(* Logix 5000 AddOnInstructionDefinition export Banner_K50Z_Param_v4; software revision 33.00 *)

TYPE Banner_IOL_Port_v4 :   // UDT that has all of the data items necessary to communicate with a specific Port on a IO-Link Master
STRUCT
   Port_Controlled : INT;   // Each bit represents a port on an IO-Link Master. Set to 1 to tell AOI to control that port.
   Port_Activate : INT;   // Each bit represents a port on an IO-Link Master. When ON that port will process any commands in queue.
   Port_Read : INT;   // Each bit represents a port on an IO-Link Master. Used to determine when device AOI has requested a Read command.
   Port_Write : INT;   // Each bit represents a port on an IO-Link Master. Used to determine when device AOI has requested a Write command.
   Port_RW_Complete : INT;   // Each bit represents a port on an IO-Link Master. Tells device AOI that Read or Write request has been completed.
   Port_Device_Read : INT;
   Data_Transfer : SINT[190];   // Array to transfer data from IO-Master to device AOIs.
END_STRUCT
END_TYPE

TYPE Banner_K50Z_BDC_v4 :   // All of the BDC data for channels 1 and 2.
STRUCT
   SP1 : DINT;   // Switchpoint.
   SP2 : DINT;   // In 2pt window mode, defines the second switching point. In other modes, SP2 is unused and must be 0.
   Switchpoint_Logic : SINT;   // 0 = Light operate, 1 = Dark operate
   BDC_Mode : INT;   // 1 = 1pt Object Set, 128 = 2pt static BGS, 129 = 2pt Window FGS, 130 = 1pt Window FGS, 131 = Dual Mode.
   Hysteresis : INT;   // A value of 0 will result in automatically calculated hysteresis.
   Delay_Mode : SINT;   // 0 = Disabled, 1 = On Off Delay, 2 = Oneshot.
   Delay_Time_On_Oneshot : DINT;   // 0 to 90000. On delay and oneshot time.
   Delay_Time_Off : DINT;   // 0 to 90000. Off delay only.
   Teach_Offset : SINT;   // 0 = Auto, 1 = User Selected
   User_Teach_Offset : DINT;   // In Object Set or Window (FGS) mode this value can be either positive or negative. In all other modes must be zero.
END_STRUCT
END_TYPE

TYPE Banner_K50Z_Pulse_Freq_v4 :
STRUCT
   Near_Freq : DINT;   // 1 to 100000 in Hz
   Far_Freq : DINT;   // 1 to 100000 in Hz
   SP1 : DINT;   // Switchpoint
   SP2 : DINT;   // In 2pt Window FGS teach, define the second switching point. In other modes SP2 should be zero.
   Pulse_Freq_LOS : DINT;   // Default value of 50. This is the Hz that the units outputs when a Loss of Signal occurs.
END_STRUCT
END_TYPE

TYPE Banner_K50Z_RD_v4 :   // UDT that stores the Write Data for a K50Z.
STRUCT
   Master_Cycle_Time : INT;
   Min_Cycle_Time : INT;
   M_Sequence_Capability : INT;
   IO_Link_Version_ID : INT;
   Process_Data_Input_Length : INT;
   Process_Data_Output_Length : INT;
   Combined_Vendor_ID : DINT;   // IO-Link Vendor ID
   Vendor_ID1 : INT;
   Vendor_ID2 : INT;
   Combined_Device_ID : DINT;   // IO-Link Device ID
   Device_ID1 : INT;
   Device_ID2 : INT;
   Device_ID3 : INT;
   Serial_Number : STRING;
   Teach_State : SINT;   // 0=Idle, 1=SP1 Success, 4=Wait for Command, 5=Busy, 7=Error.
   SP1_TP1 : SINT;
   SP1_TP2 : SINT;
   Measurement_Z1 : DINT;
   Excess_Gain_Z1 : DINT;   // Amount of singal measured over the minimum threshold.
   Stability_Z1 : SINT;   // 0=No target exists, 1=Marginal signal, 2=Stable.
   Measurement_Z2 : DINT;
   Excess_Gain_Z2 : DINT;   // Amount of singal measured over the minimum threshold.
   Stability_Z2 : SINT;   // 0=No target exists, 1=Marginal signal, 2=Stable.
   Emitter_Status : SINT;   // 0 = Active, 1 = Inactive
   Temperature : DINT;   // Internal temperature measurement for the device.
   Last_Taught_Temperature : DINT;   // Internal Temperature the last time device was taught.
   MDC_Lower_Limit : DINT;
   MDC_Upper_Limit : DINT;
   MDC_Unit : INT;
   MDC_Scale : SINT;
END_STRUCT
END_TYPE

TYPE Banner_K50Z_v4 :   // All of the parameters for a K50Z.
STRUCT
   Initial_Global_Read : BOOL;   // Determines if all of the IO-Link data has been read into the PLC yet
   Command : INT;   // Value placed in here will activate a read or write to a specifc IO-Link Index
   Read : Banner_K50Z_RD_v4;   // Read Only Data
   Write : Banner_K50Z_WD_v4;   // Write Data
   Archive : Banner_K50Z_WD_v4;   // Archive Data
   Reset : BOOL;   // Resets AOI. This will force a complete parameter read of the sensor.
END_STRUCT
END_TYPE

TYPE Banner_K50Z_WD_v4 :   // UDT that stores the Write Data for a K50Z.
STRUCT
   System_Command : INT;   // See IODD file for list of commands that can be activated via the System Command interface
   Parameter_Access_Lock : SINT;   // Write access to all parameters is prohibited while value is 1. Only this parameter can be adjusted when value is 1.
   Data_Storage_Lock : SINT;   // Automatic data storage is disabled when this value is equal to 1. Read access is not affected.
   Local_Parameterization_Lock : SINT;   // Parameterization via local control elements on device is disabled.
   Local_User_Interface_Lock : SINT;   // Operation of local user interface is disabled.
   Teach_Channel : SINT;   // 0 = Default, 1 = BDC1, 2 = BDC2
   Response_Speed : SINT;   // 0 = Speed 0, 1 = Speed 1, 2 = Speed 2, 3 = Speed 3
   Remote_Input_Mode : SINT;   // 0 = Remote Teach Input, 1 = Emitter On, 2 = Emitter Off
   Secondary_Output_Mode : SINT;   // 0 = Independent Output, 1 = Complementary Output, 2 = Pulse Frequency Output
   IOL_Filter_Time : INT;   // Time to average IOl process data measurement between updates
   Include_Binary : SINT;   // 0 = Include, 1 = Don't Include, 2= Measurement Device
   Measurement_1 : SINT;   // 0 = Disabled, 1 = Excess Gain Z1, 2 = Excess Gain Z2, 3 = Excess Gain / 10 Z1, 4 = Excess Gain / 10 Z2, 5 = Measurement Z1, 6 = Measurement Z2.
   Measurement_2 : SINT;   // 0 = Disabled, 1 = Excess Gain Z1, 2 = Excess Gain Z2, 3 = Excess Gain / 10 Z1, 4 = Excess Gain / 10 Z2, 5 = Measurement Z1, 6 = Measurement Z2.
   Digital_Measuring_Sensor_Zone_Selection : SINT;   // 0=Zone 1, 1=Zone2
   BDC : Banner_K50Z_BDC_v4[3];
   Pulse_Freq : Banner_K50Z_Pulse_Freq_v4;
END_STRUCT
END_TYPE

ADD_ON_INSTRUCTION Banner_K50Z_Param_v4   (* revision 4.1, vendor Banner Engineering *)
// AOI to read and write parameter data to an IO-Link K50Z.
VAR_IN_OUT
   K50Z : Banner_K50Z_v4; {required}
   Port_Data : Banner_IOL_Port_v4; {required}
END_VAR
VAR_INPUT
   Port : DINT; {required}
END_VAR
VAR
   Local_Control : DINT; {access None}
   Global_Read_Command_Value : INT; {access None}
   Global_Write_Command_Value : INT; {access None}
   Command_Being_Processed : BOOL; {access None}
   Update_Archive : BOOL; {access None}
   Index_Write_Inprocess : INT; {access None}
   Index_Write_Control : INT; {access None}
   Inprocess_Index : DINT; {access None}
END_VAR

ROUTINE Logic   (* ladder *)
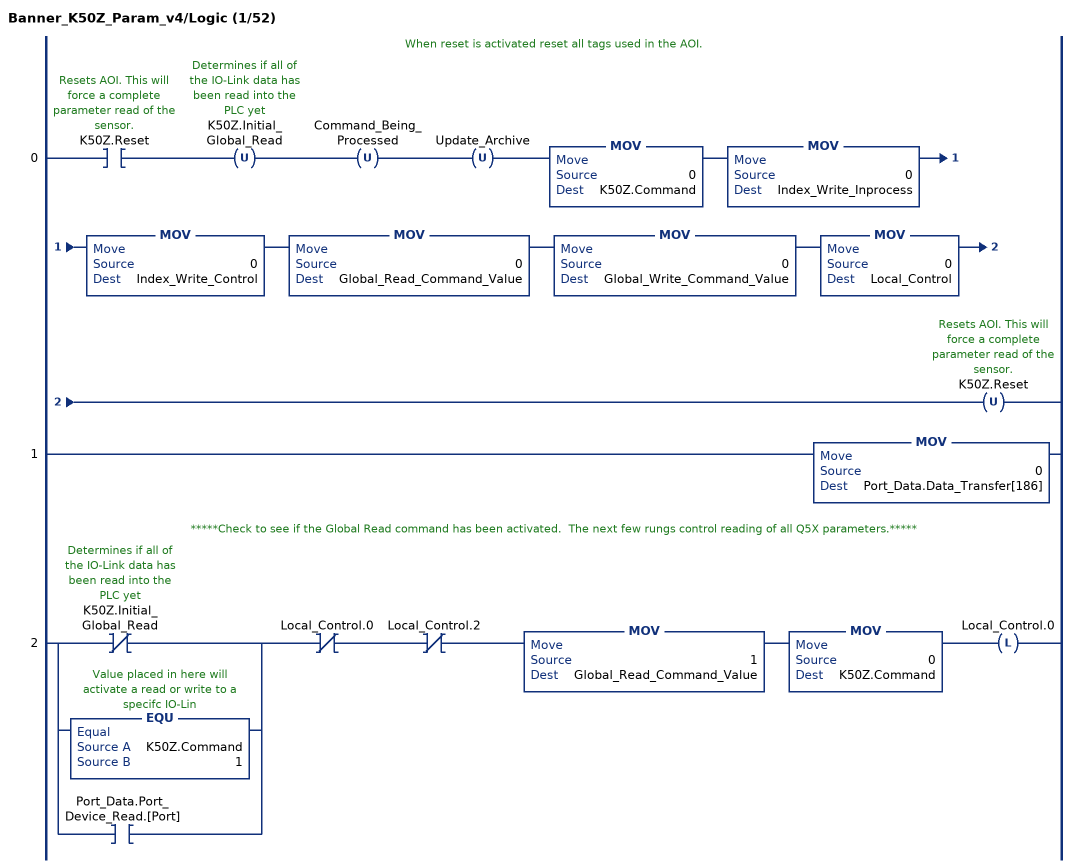
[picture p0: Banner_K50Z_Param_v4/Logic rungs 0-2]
   // When reset is activated reset all tags used in the AOI.
   0: XIC(K50Z.Reset)OTU(K50Z.Initial_Global_Read)OTU(Command_Being_Processed)OTU(Update_Archive)MOV(0,K50Z.Command)MOV(0,Index_Write_Inprocess)MOV(0,Index_Write_Control)MOV(0,Global_Read_Command_Value)MOV(0,Global_Write_Command_Value)MOV(0,Local_Control)OTU(K50Z.Reset);
   1: MOV(0,Port_Data.Data_Transfer[186]);
   // *****Check to see if the Global Read command has been activated.  The next few rungs control reading of all Q5X parameters.*****
   2: [XIO(K50Z.Initial_Global_Read) ,EQU(K50Z.Command,1) ,XIC(Port_Data.Port_Device_Read.[Port]) ]XIO(Local_Control.0)XIO(Local_Control.2)MOV(1,Global_Read_Command_Value)MOV(0,K50Z.Command)OTL(Local_Control.0);
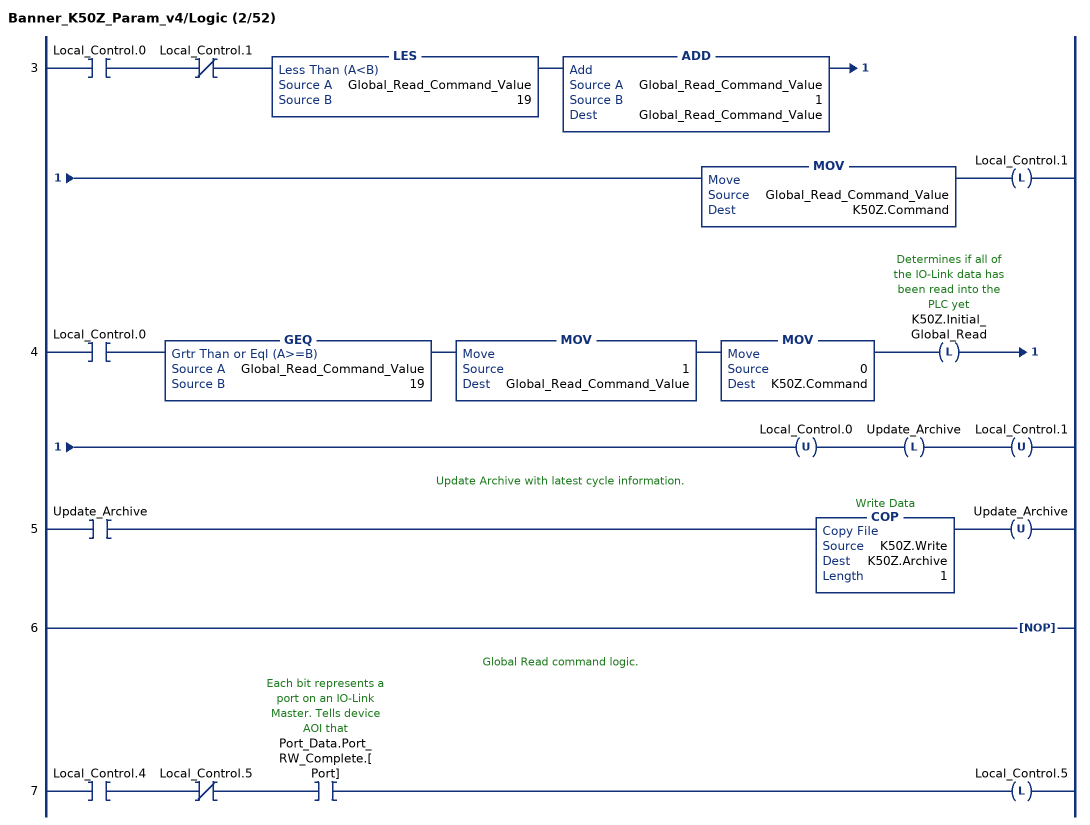
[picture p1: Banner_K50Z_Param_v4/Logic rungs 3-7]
   3: XIC(Local_Control.0)XIO(Local_Control.1)LES(Global_Read_Command_Value,19)ADD(Global_Read_Command_Value,1,Global_Read_Command_Value)MOV(Global_Read_Command_Value,K50Z.Command)OTL(Local_Control.1);
   4: XIC(Local_Control.0)GEQ(Global_Read_Command_Value,19)MOV(1,Global_Read_Command_Value)MOV(0,K50Z.Command)OTL(K50Z.Initial_Global_Read)OTU(Local_Control.0)OTL(Update_Archive)OTU(Local_Control.1);
   // Update Archive with latest cycle information.
   5: XIC(Update_Archive)COP(K50Z.Write,K50Z.Archive,1)OTU(Update_Archive);
   6: NOP();
   // Global Read command logic.
   7: XIC(Local_Control.4)XIO(Local_Control.5)XIC(Port_Data.Port_RW_Complete.[Port])OTL(Local_Control.5);
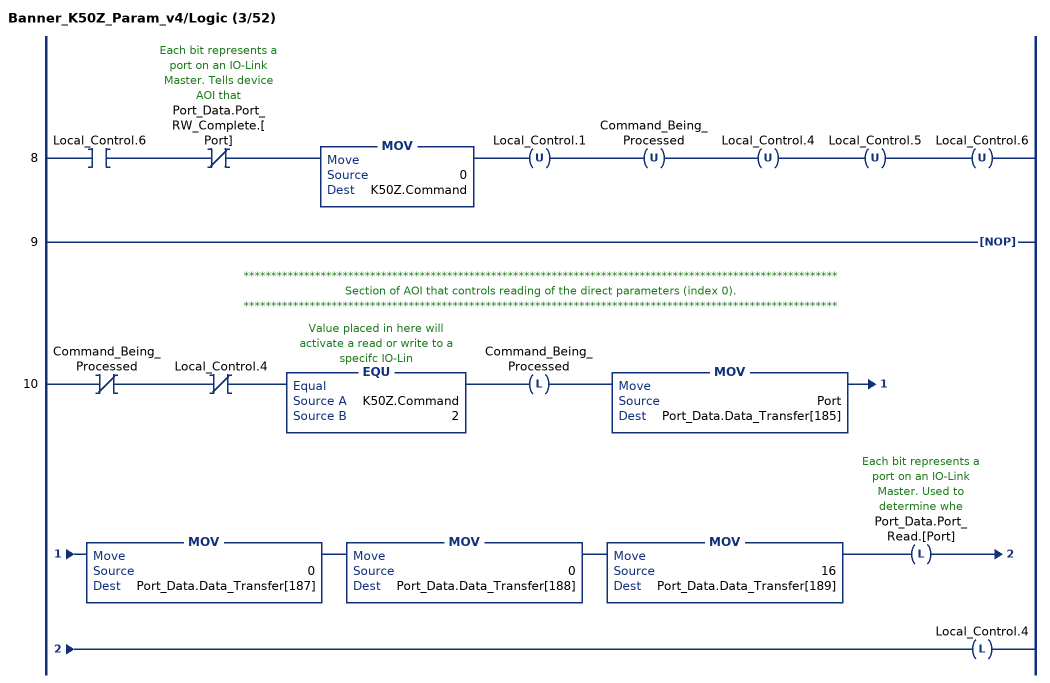
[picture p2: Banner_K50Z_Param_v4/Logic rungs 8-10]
   8: XIC(Local_Control.6)XIO(Port_Data.Port_RW_Complete.[Port])MOV(0,K50Z.Command)OTU(Local_Control.1)OTU(Command_Being_Processed)OTU(Local_Control.4)OTU(Local_Control.5)OTU(Local_Control.6);
   9: NOP();
   // ************************************************************************************************************
   // Section of AOI that controls reading of the direct parameters (index 0).
   // ************************************************************************************************************
   10: XIO(Command_Being_Processed)XIO(Local_Control.4)EQU(K50Z.Command,2)OTL(Command_Being_Processed)MOV(Port,Port_Data.Data_Transfer[185])MOV(0,Port_Data.Data_Transfer[187])MOV(0,Port_Data.Data_Transfer[188])MOV(16,Port_Data.Data_Transfer[189])OTL(Port_Data.Port_Read.[Port])OTL(Local_Control.4);
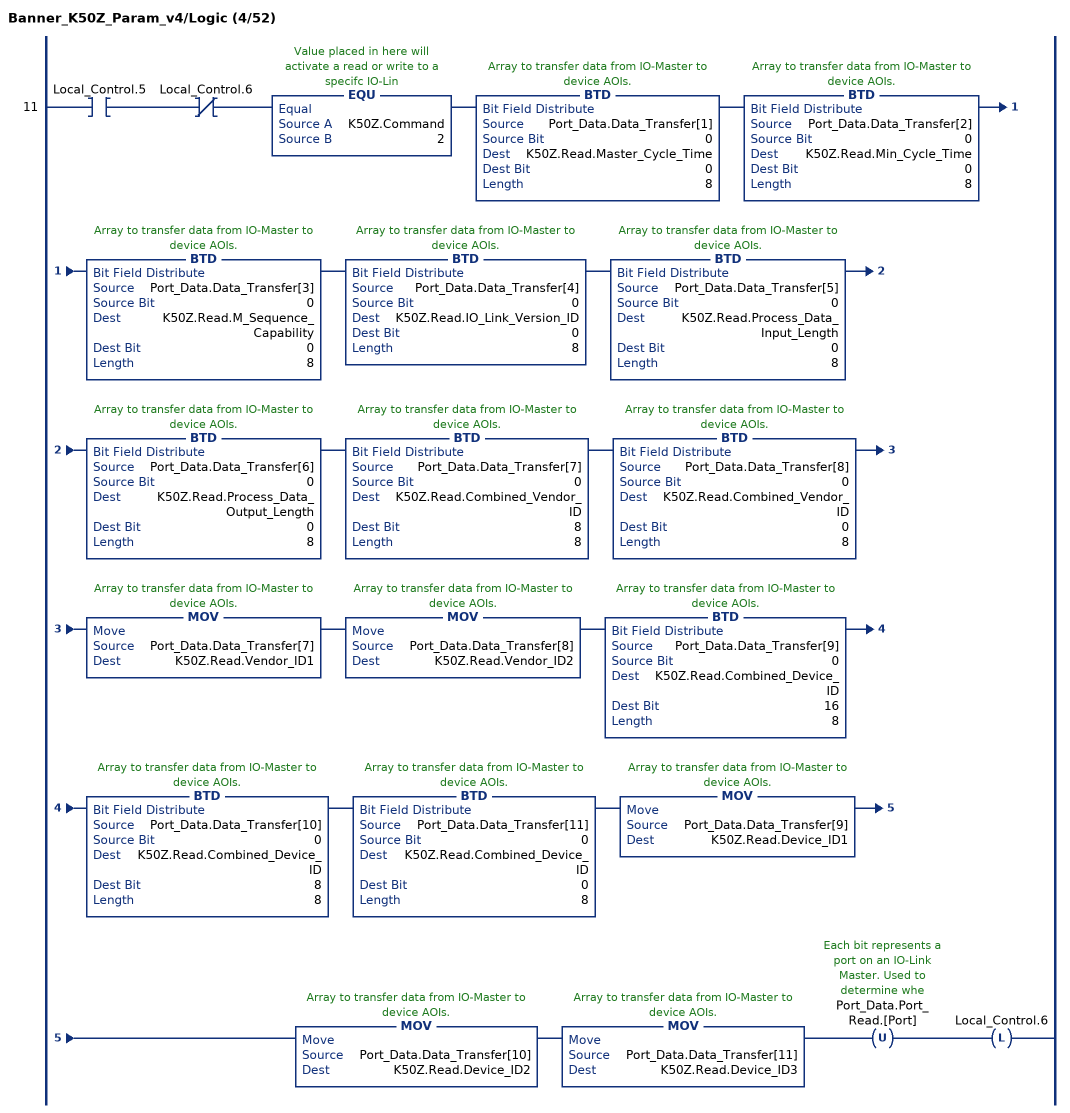
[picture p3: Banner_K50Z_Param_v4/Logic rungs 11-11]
   11: XIC(Local_Control.5)XIO(Local_Control.6)EQU(K50Z.Command,2)BTD(Port_Data.Data_Transfer[1],0,K50Z.Read.Master_Cycle_Time,0,8)BTD(Port_Data.Data_Transfer[2],0,K50Z.Read.Min_Cycle_Time,0,8)BTD(Port_Data.Data_Transfer[3],0,K50Z.Read.M_Sequence_Capability,0,8)BTD(Port_Data.Data_Transfer[4],0,K50Z.Read.IO_Link_Version_ID,0,8)BTD(Port_Data.Data_Transfer[5],0,K50Z.Read.Process_Data_Input_Length,0,8)BTD(Port_Data.Data_Transfer[6],0,K50Z.Read.Process_Data_Output_Length,0,8)BTD(Port_Data.Data_Transfer[7],0,K50Z.Read.Combined_Vendor_ID,8,8)BTD(Port_Data.Data_Transfer[8],0,K50Z.Read.Combined_Vendor_ID,0,8)MOV(Port_Data.Data_Transfer[7],K50Z.Read.Vendor_ID1)MOV(Port_Data.Data_Transfer[8],K50Z.Read.Vendor_ID2)BTD(Port_Data.Data_Transfer[9],0,K50Z.Read.Combined_Device_ID,16,8)BTD(Port_Data.Data_Transfer[10],0,K50Z.Read.Combined_Device_ID,8,8)BTD(Port_Data.Data_Transfer[11],0,K50Z.Read.Combined_Device_ID,0,8)MOV(Port_Data.Data_Transfer[9],K50Z.Read.Device_ID1)MOV(Port_Data.Data_Transfer[10],K50Z.Read.Device_ID2)MOV(Port_Data.Data_Transfer[11],K50Z.Read.Device_ID3)OTU(Port_Data.Port_Read.[Port])OTL(Local_Control.6);
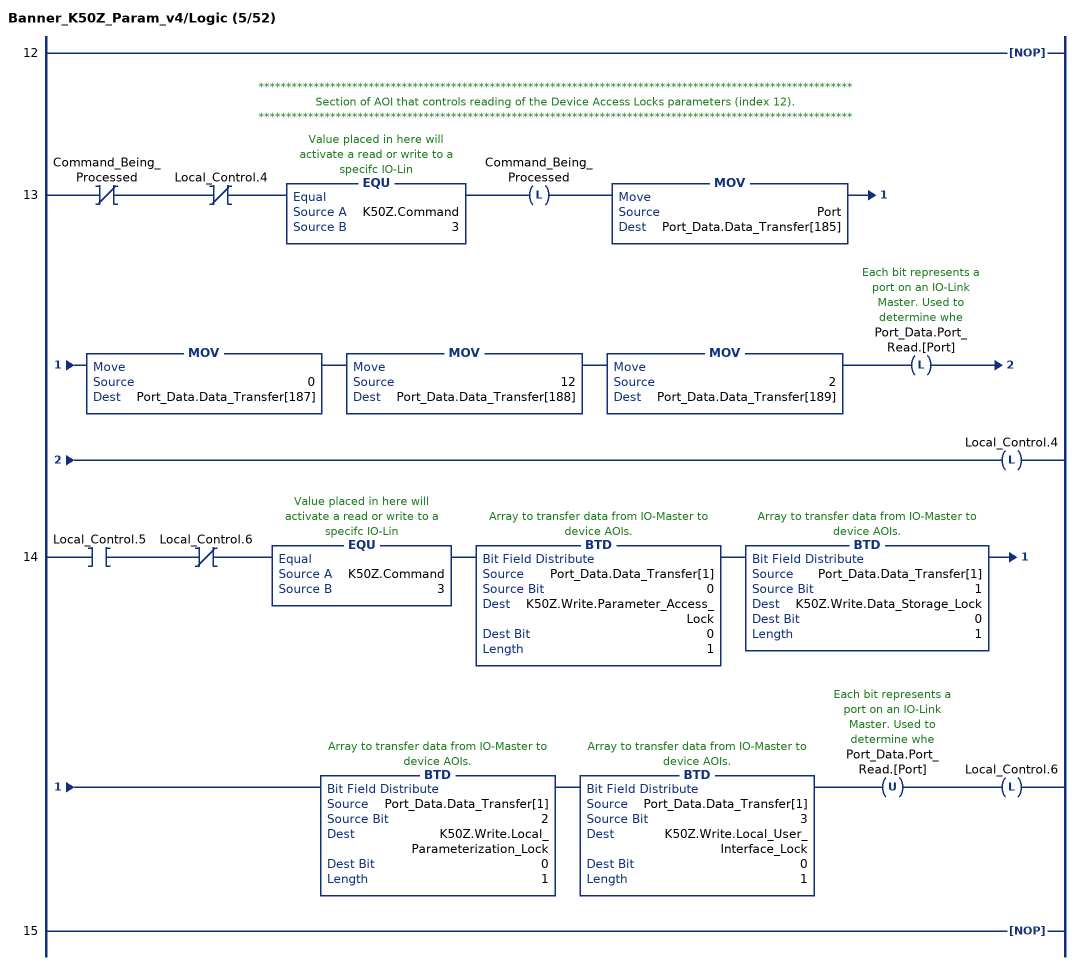
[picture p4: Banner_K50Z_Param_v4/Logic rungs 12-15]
   12: NOP();
   // ************************************************************************************************************
   // Section of AOI that controls reading of the Device Access Locks parameters (index 12).
   // ************************************************************************************************************
   13: XIO(Command_Being_Processed)XIO(Local_Control.4)EQU(K50Z.Command,3)OTL(Command_Being_Processed)MOV(Port,Port_Data.Data_Transfer[185])MOV(0,Port_Data.Data_Transfer[187])MOV(12,Port_Data.Data_Transfer[188])MOV(2,Port_Data.Data_Transfer[189])OTL(Port_Data.Port_Read.[Port])OTL(Local_Control.4);
   14: XIC(Local_Control.5)XIO(Local_Control.6)EQU(K50Z.Command,3)BTD(Port_Data.Data_Transfer[1],0,K50Z.Write.Parameter_Access_Lock,0,1)BTD(Port_Data.Data_Transfer[1],1,K50Z.Write.Data_Storage_Lock,0,1)BTD(Port_Data.Data_Transfer[1],2,K50Z.Write.Local_Parameterization_Lock,0,1)BTD(Port_Data.Data_Transfer[1],3,K50Z.Write.Local_User_Interface_Lock,0,1)OTU(Port_Data.Port_Read.[Port])OTL(Local_Control.6);
   15: NOP();
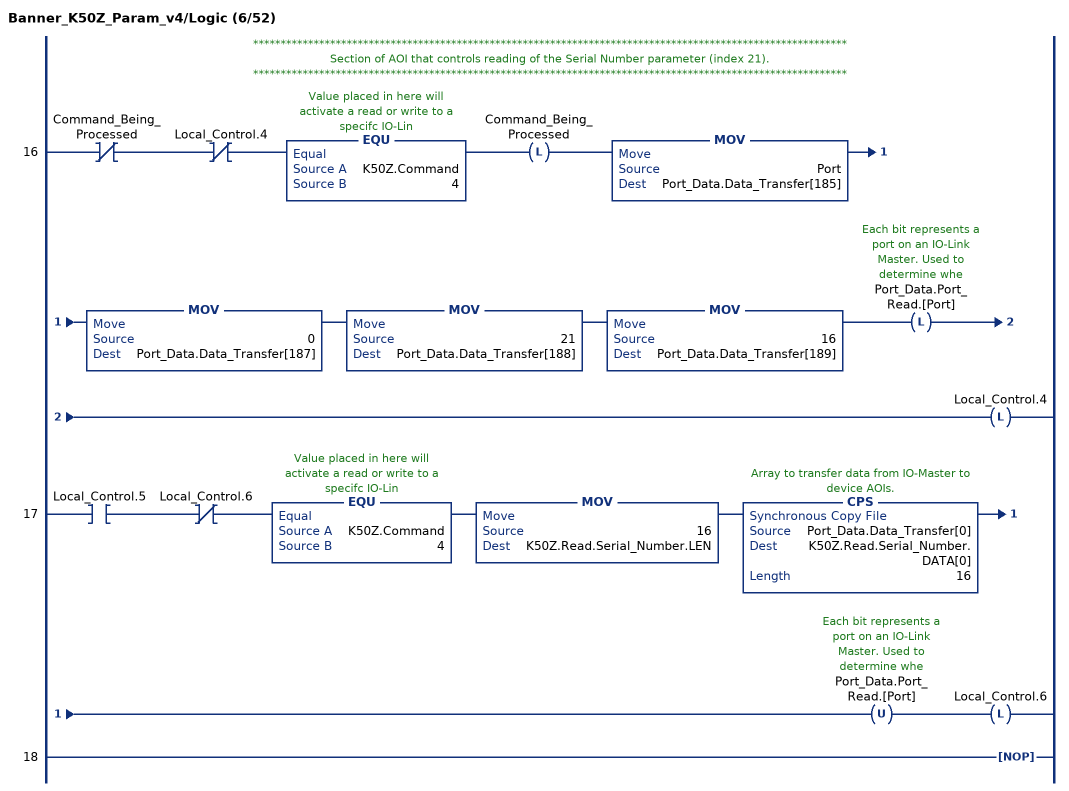
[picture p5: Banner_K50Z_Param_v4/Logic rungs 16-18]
   // ************************************************************************************************************
   // Section of AOI that controls reading of the Serial Number parameter (index 21).
   // ************************************************************************************************************
   16: XIO(Command_Being_Processed)XIO(Local_Control.4)EQU(K50Z.Command,4)OTL(Command_Being_Processed)MOV(Port,Port_Data.Data_Transfer[185])MOV(0,Port_Data.Data_Transfer[187])MOV(21,Port_Data.Data_Transfer[188])MOV(16,Port_Data.Data_Transfer[189])OTL(Port_Data.Port_Read.[Port])OTL(Local_Control.4);
   17: XIC(Local_Control.5)XIO(Local_Control.6)EQU(K50Z.Command,4)MOV(16,K50Z.Read.Serial_Number.LEN)CPS(Port_Data.Data_Transfer[0],K50Z.Read.Serial_Number.DATA[0],16)OTU(Port_Data.Port_Read.[Port])OTL(Local_Control.6);
   18: NOP();
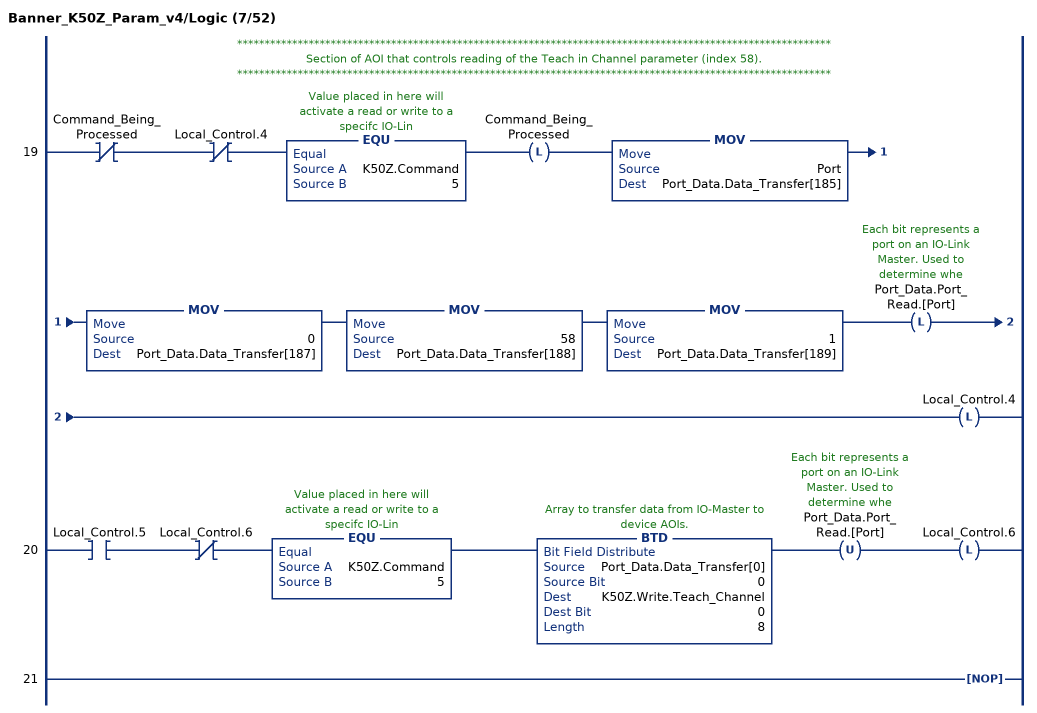
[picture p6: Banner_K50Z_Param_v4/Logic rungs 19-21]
   // ************************************************************************************************************
   // Section of AOI that controls reading of the Teach in Channel parameter (index 58).
   // ************************************************************************************************************
   19: XIO(Command_Being_Processed)XIO(Local_Control.4)EQU(K50Z.Command,5)OTL(Command_Being_Processed)MOV(Port,Port_Data.Data_Transfer[185])MOV(0,Port_Data.Data_Transfer[187])MOV(58,Port_Data.Data_Transfer[188])MOV(1,Port_Data.Data_Transfer[189])OTL(Port_Data.Port_Read.[Port])OTL(Local_Control.4);
   20: XIC(Local_Control.5)XIO(Local_Control.6)EQU(K50Z.Command,5)BTD(Port_Data.Data_Transfer[0],0,K50Z.Write.Teach_Channel,0,8)OTU(Port_Data.Port_Read.[Port])OTL(Local_Control.6);
   21: NOP();
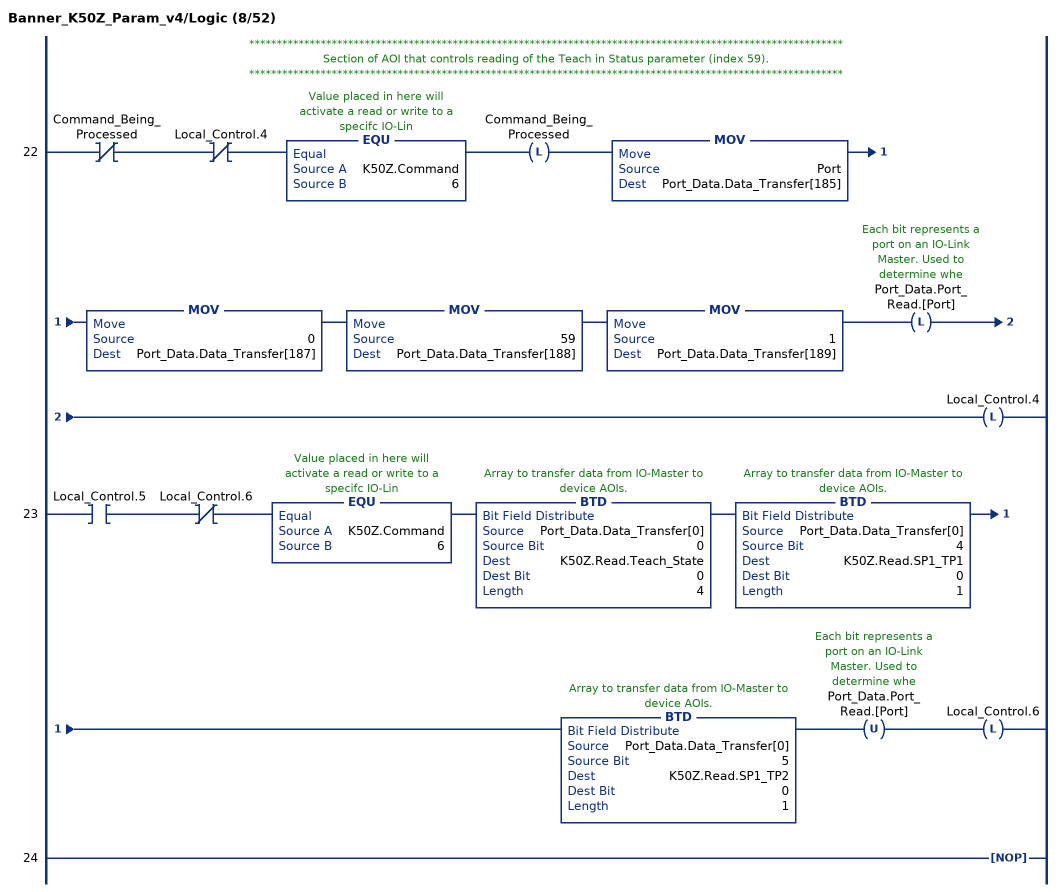
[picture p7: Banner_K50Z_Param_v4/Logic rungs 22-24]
   // ************************************************************************************************************
   // Section of AOI that controls reading of the Teach in Status parameter (index 59).
   // ************************************************************************************************************
   22: XIO(Command_Being_Processed)XIO(Local_Control.4)EQU(K50Z.Command,6)OTL(Command_Being_Processed)MOV(Port,Port_Data.Data_Transfer[185])MOV(0,Port_Data.Data_Transfer[187])MOV(59,Port_Data.Data_Transfer[188])MOV(1,Port_Data.Data_Transfer[189])OTL(Port_Data.Port_Read.[Port])OTL(Local_Control.4);
   23: XIC(Local_Control.5)XIO(Local_Control.6)EQU(K50Z.Command,6)BTD(Port_Data.Data_Transfer[0],0,K50Z.Read.Teach_State,0,4)BTD(Port_Data.Data_Transfer[0],4,K50Z.Read.SP1_TP1,0,1)BTD(Port_Data.Data_Transfer[0],5,K50Z.Read.SP1_TP2,0,1)OTU(Port_Data.Port_Read.[Port])OTL(Local_Control.6);
   24: NOP();
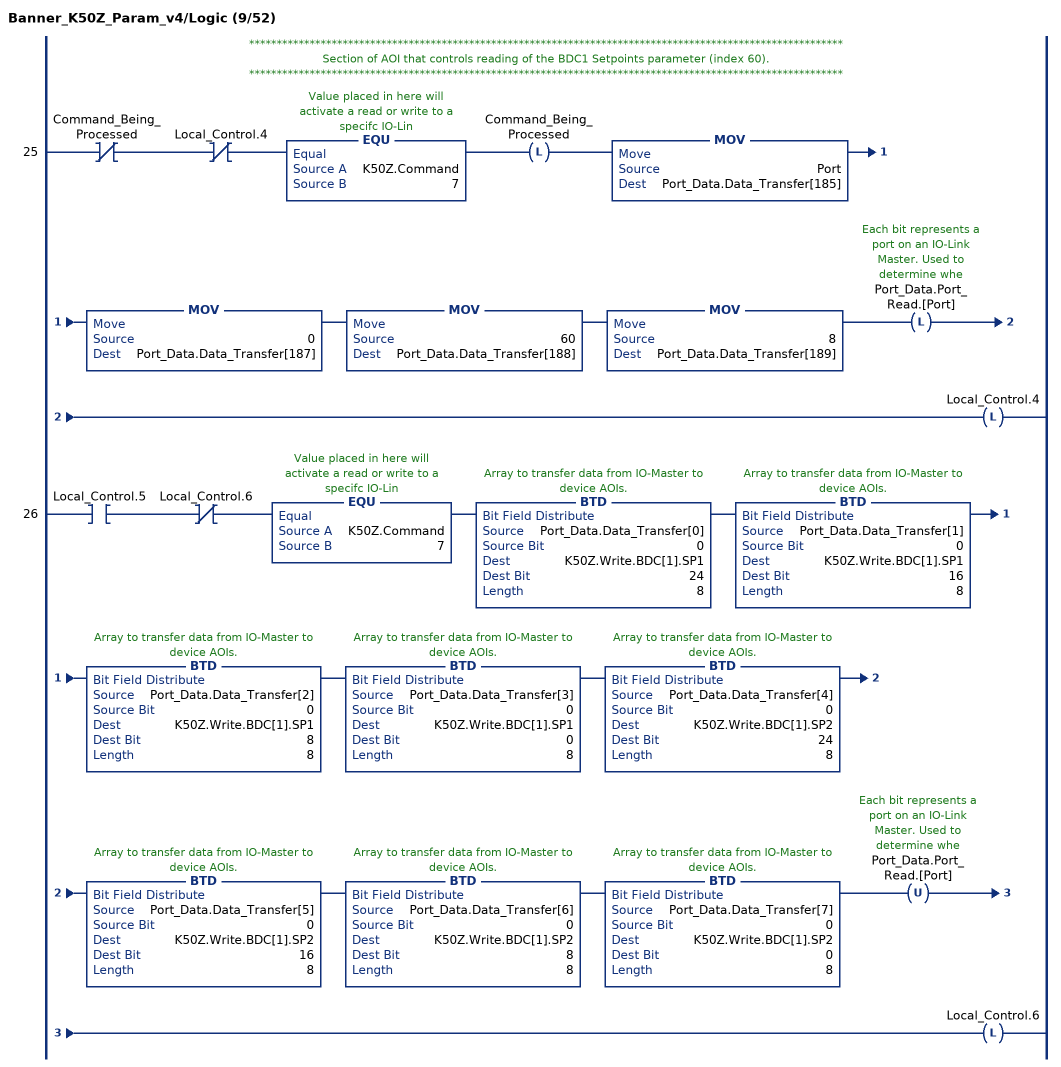
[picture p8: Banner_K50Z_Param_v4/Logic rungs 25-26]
   // ************************************************************************************************************
   // Section of AOI that controls reading of the BDC1 Setpoints parameter (index 60).
   // ************************************************************************************************************
   25: XIO(Command_Being_Processed)XIO(Local_Control.4)EQU(K50Z.Command,7)OTL(Command_Being_Processed)MOV(Port,Port_Data.Data_Transfer[185])MOV(0,Port_Data.Data_Transfer[187])MOV(60,Port_Data.Data_Transfer[188])MOV(8,Port_Data.Data_Transfer[189])OTL(Port_Data.Port_Read.[Port])OTL(Local_Control.4);
   26: XIC(Local_Control.5)XIO(Local_Control.6)EQU(K50Z.Command,7)BTD(Port_Data.Data_Transfer[0],0,K50Z.Write.BDC[1].SP1,24,8)BTD(Port_Data.Data_Transfer[1],0,K50Z.Write.BDC[1].SP1,16,8)BTD(Port_Data.Data_Transfer[2],0,K50Z.Write.BDC[1].SP1,8,8)BTD(Port_Data.Data_Transfer[3],0,K50Z.Write.BDC[1].SP1,0,8)BTD(Port_Data.Data_Transfer[4],0,K50Z.Write.BDC[1].SP2,24,8)BTD(Port_Data.Data_Transfer[5],0,K50Z.Write.BDC[1].SP2,16,8)BTD(Port_Data.Data_Transfer[6],0,K50Z.Write.BDC[1].SP2,8,8)BTD(Port_Data.Data_Transfer[7],0,K50Z.Write.BDC[1].SP2,0,8)OTU(Port_Data.Port_Read.[Port])OTL(Local_Control.6);
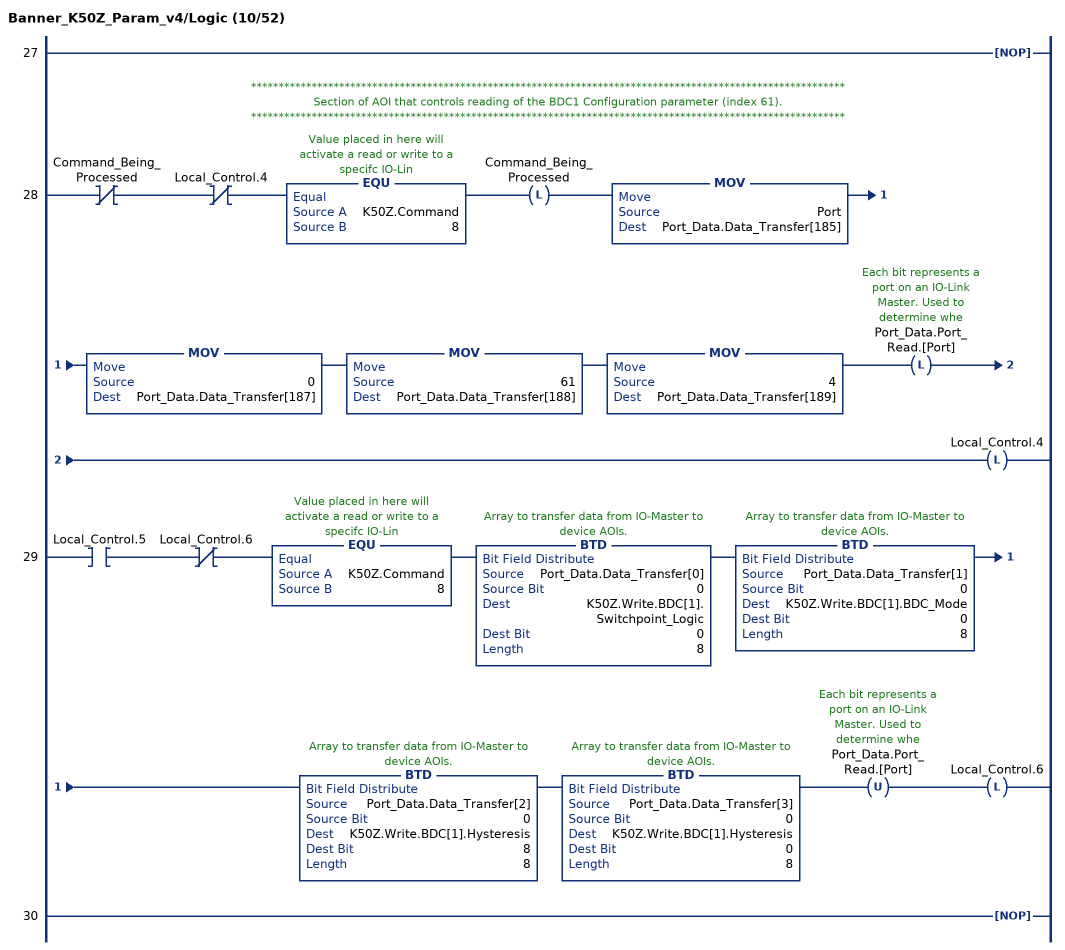
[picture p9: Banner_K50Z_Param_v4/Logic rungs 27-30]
   27: NOP();
   // ************************************************************************************************************
   // Section of AOI that controls reading of the BDC1 Configuration parameter (index 61).
   // ************************************************************************************************************
   28: XIO(Command_Being_Processed)XIO(Local_Control.4)EQU(K50Z.Command,8)OTL(Command_Being_Processed)MOV(Port,Port_Data.Data_Transfer[185])MOV(0,Port_Data.Data_Transfer[187])MOV(61,Port_Data.Data_Transfer[188])MOV(4,Port_Data.Data_Transfer[189])OTL(Port_Data.Port_Read.[Port])OTL(Local_Control.4);
   29: XIC(Local_Control.5)XIO(Local_Control.6)EQU(K50Z.Command,8)BTD(Port_Data.Data_Transfer[0],0,K50Z.Write.BDC[1].Switchpoint_Logic,0,8)BTD(Port_Data.Data_Transfer[1],0,K50Z.Write.BDC[1].BDC_Mode,0,8)BTD(Port_Data.Data_Transfer[2],0,K50Z.Write.BDC[1].Hysteresis,8,8)BTD(Port_Data.Data_Transfer[3],0,K50Z.Write.BDC[1].Hysteresis,0,8)OTU(Port_Data.Port_Read.[Port])OTL(Local_Control.6);
   30: NOP();
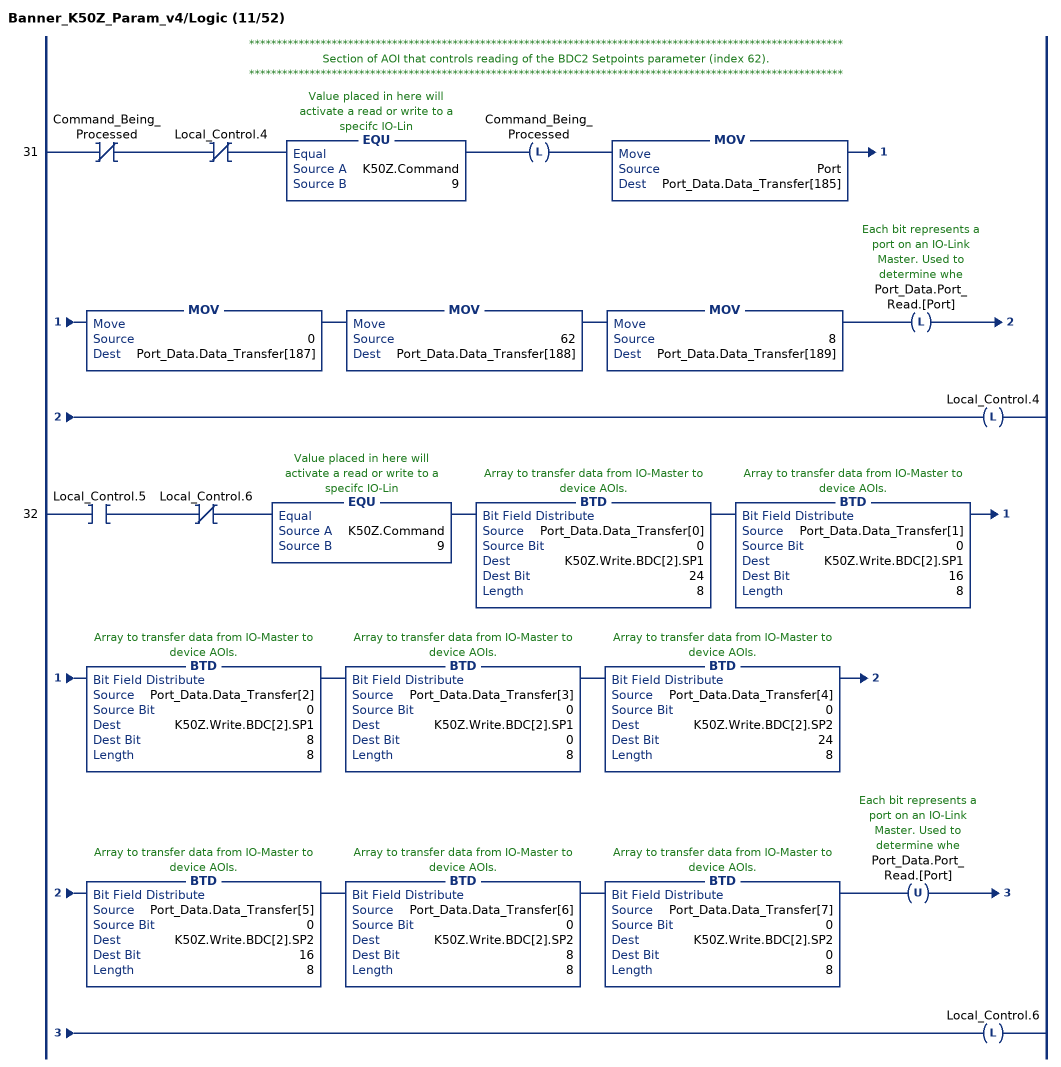
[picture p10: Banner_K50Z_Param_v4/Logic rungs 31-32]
   // ************************************************************************************************************
   // Section of AOI that controls reading of the BDC2 Setpoints parameter (index 62).
   // ************************************************************************************************************
   31: XIO(Command_Being_Processed)XIO(Local_Control.4)EQU(K50Z.Command,9)OTL(Command_Being_Processed)MOV(Port,Port_Data.Data_Transfer[185])MOV(0,Port_Data.Data_Transfer[187])MOV(62,Port_Data.Data_Transfer[188])MOV(8,Port_Data.Data_Transfer[189])OTL(Port_Data.Port_Read.[Port])OTL(Local_Control.4);
   32: XIC(Local_Control.5)XIO(Local_Control.6)EQU(K50Z.Command,9)BTD(Port_Data.Data_Transfer[0],0,K50Z.Write.BDC[2].SP1,24,8)BTD(Port_Data.Data_Transfer[1],0,K50Z.Write.BDC[2].SP1,16,8)BTD(Port_Data.Data_Transfer[2],0,K50Z.Write.BDC[2].SP1,8,8)BTD(Port_Data.Data_Transfer[3],0,K50Z.Write.BDC[2].SP1,0,8)BTD(Port_Data.Data_Transfer[4],0,K50Z.Write.BDC[2].SP2,24,8)BTD(Port_Data.Data_Transfer[5],0,K50Z.Write.BDC[2].SP2,16,8)BTD(Port_Data.Data_Transfer[6],0,K50Z.Write.BDC[2].SP2,8,8)BTD(Port_Data.Data_Transfer[7],0,K50Z.Write.BDC[2].SP2,0,8)OTU(Port_Data.Port_Read.[Port])OTL(Local_Control.6);
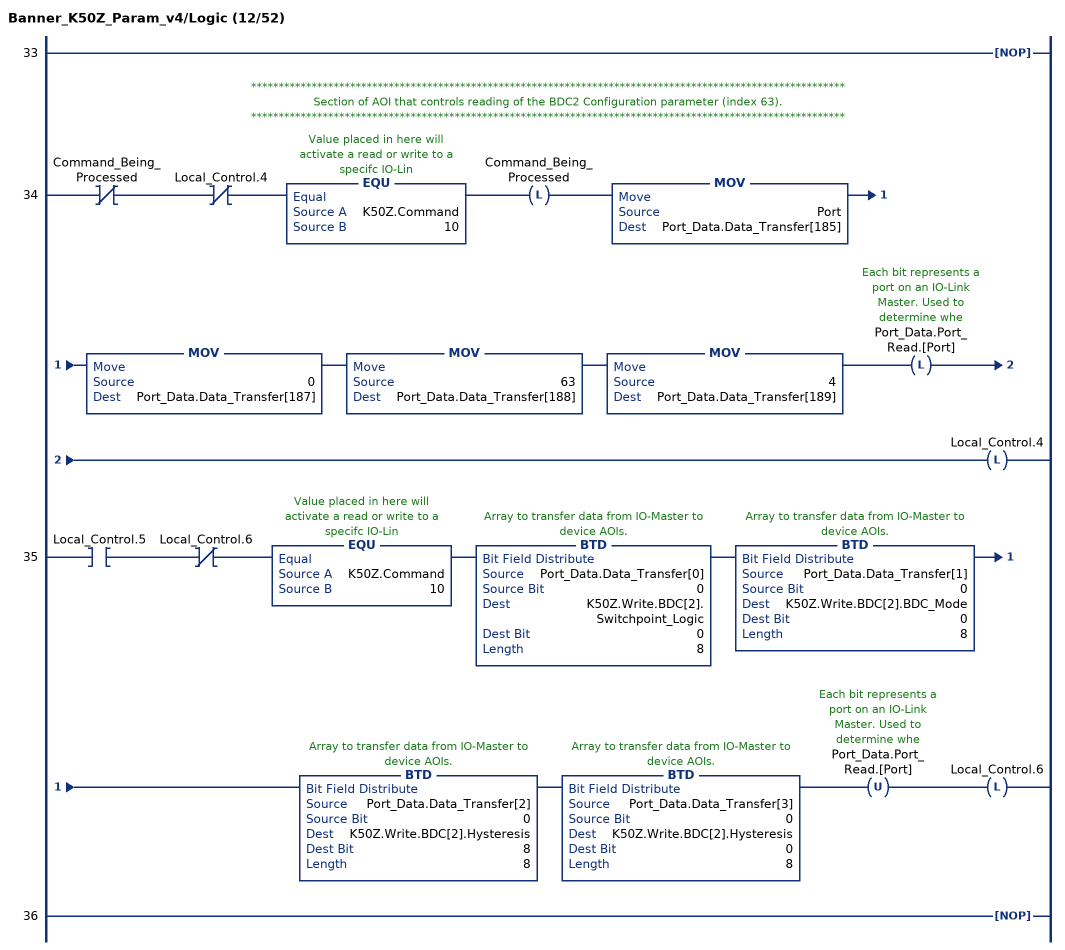
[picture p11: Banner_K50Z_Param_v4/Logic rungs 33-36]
   33: NOP();
   // ************************************************************************************************************
   // Section of AOI that controls reading of the BDC2 Configuration parameter (index 63).
   // ************************************************************************************************************
   34: XIO(Command_Being_Processed)XIO(Local_Control.4)EQU(K50Z.Command,10)OTL(Command_Being_Processed)MOV(Port,Port_Data.Data_Transfer[185])MOV(0,Port_Data.Data_Transfer[187])MOV(63,Port_Data.Data_Transfer[188])MOV(4,Port_Data.Data_Transfer[189])OTL(Port_Data.Port_Read.[Port])OTL(Local_Control.4);
   35: XIC(Local_Control.5)XIO(Local_Control.6)EQU(K50Z.Command,10)BTD(Port_Data.Data_Transfer[0],0,K50Z.Write.BDC[2].Switchpoint_Logic,0,8)BTD(Port_Data.Data_Transfer[1],0,K50Z.Write.BDC[2].BDC_Mode,0,8)BTD(Port_Data.Data_Transfer[2],0,K50Z.Write.BDC[2].Hysteresis,8,8)BTD(Port_Data.Data_Transfer[3],0,K50Z.Write.BDC[2].Hysteresis,0,8)OTU(Port_Data.Port_Read.[Port])OTL(Local_Control.6);
   36: NOP();
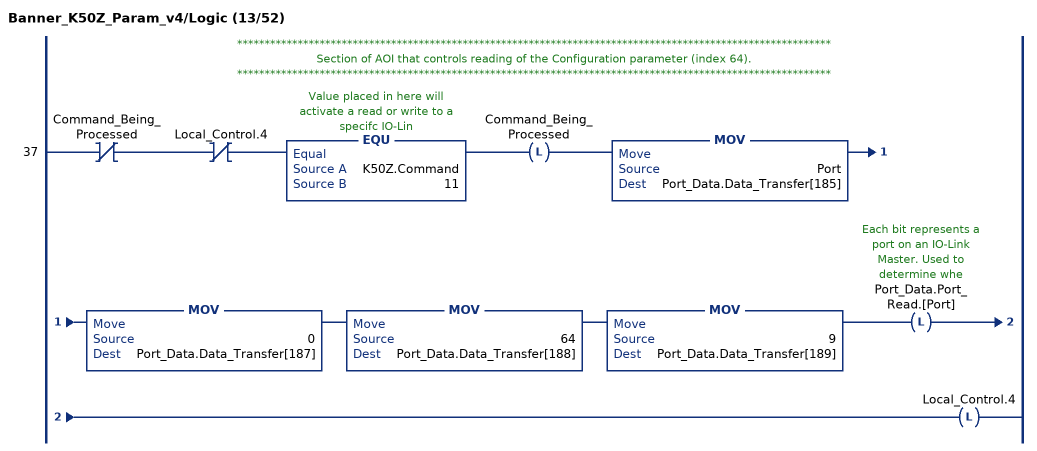
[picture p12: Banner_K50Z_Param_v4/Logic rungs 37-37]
   // ************************************************************************************************************
   // Section of AOI that controls reading of the Configuration parameter (index 64).
   // ************************************************************************************************************
   37: XIO(Command_Being_Processed)XIO(Local_Control.4)EQU(K50Z.Command,11)OTL(Command_Being_Processed)MOV(Port,Port_Data.Data_Transfer[185])MOV(0,Port_Data.Data_Transfer[187])MOV(64,Port_Data.Data_Transfer[188])MOV(9,Port_Data.Data_Transfer[189])OTL(Port_Data.Port_Read.[Port])OTL(Local_Control.4);
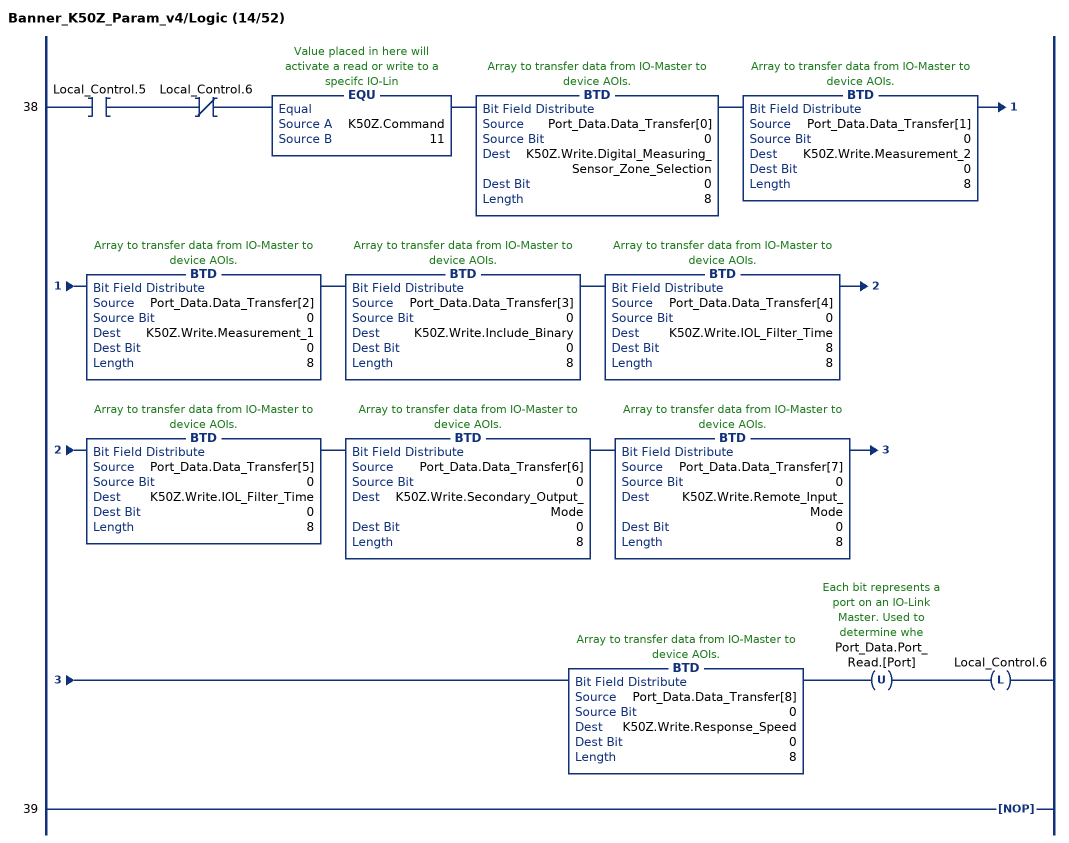
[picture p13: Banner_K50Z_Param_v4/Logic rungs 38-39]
   38: XIC(Local_Control.5)XIO(Local_Control.6)EQU(K50Z.Command,11)BTD(Port_Data.Data_Transfer[0],0,K50Z.Write.Digital_Measuring_Sensor_Zone_Selection,0,8)BTD(Port_Data.Data_Transfer[1],0,K50Z.Write.Measurement_2,0,8)BTD(Port_Data.Data_Transfer[2],0,K50Z.Write.Measurement_1,0,8)BTD(Port_Data.Data_Transfer[3],0,K50Z.Write.Include_Binary,0,8)BTD(Port_Data.Data_Transfer[4],0,K50Z.Write.IOL_Filter_Time,8,8)BTD(Port_Data.Data_Transfer[5],0,K50Z.Write.IOL_Filter_Time,0,8)BTD(Port_Data.Data_Transfer[6],0,K50Z.Write.Secondary_Output_Mode,0,8)BTD(Port_Data.Data_Transfer[7],0,K50Z.Write.Remote_Input_Mode,0,8)BTD(Port_Data.Data_Transfer[8],0,K50Z.Write.Response_Speed,0,8)OTU(Port_Data.Port_Read.[Port])OTL(Local_Control.6);
   39: NOP();
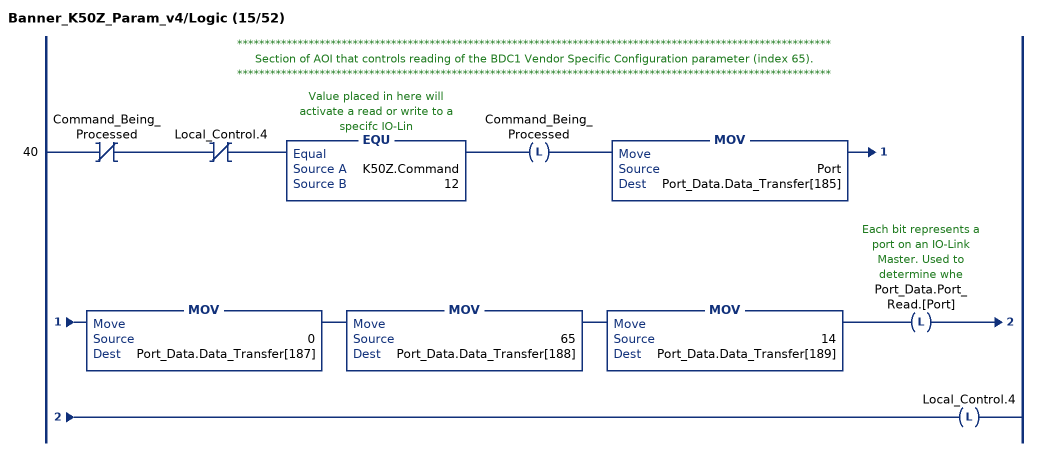
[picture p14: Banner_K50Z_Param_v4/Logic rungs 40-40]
   // ************************************************************************************************************
   // Section of AOI that controls reading of the BDC1 Vendor Specific Configuration parameter (index 65).
   // ************************************************************************************************************
   40: XIO(Command_Being_Processed)XIO(Local_Control.4)EQU(K50Z.Command,12)OTL(Command_Being_Processed)MOV(Port,Port_Data.Data_Transfer[185])MOV(0,Port_Data.Data_Transfer[187])MOV(65,Port_Data.Data_Transfer[188])MOV(14,Port_Data.Data_Transfer[189])OTL(Port_Data.Port_Read.[Port])OTL(Local_Control.4);
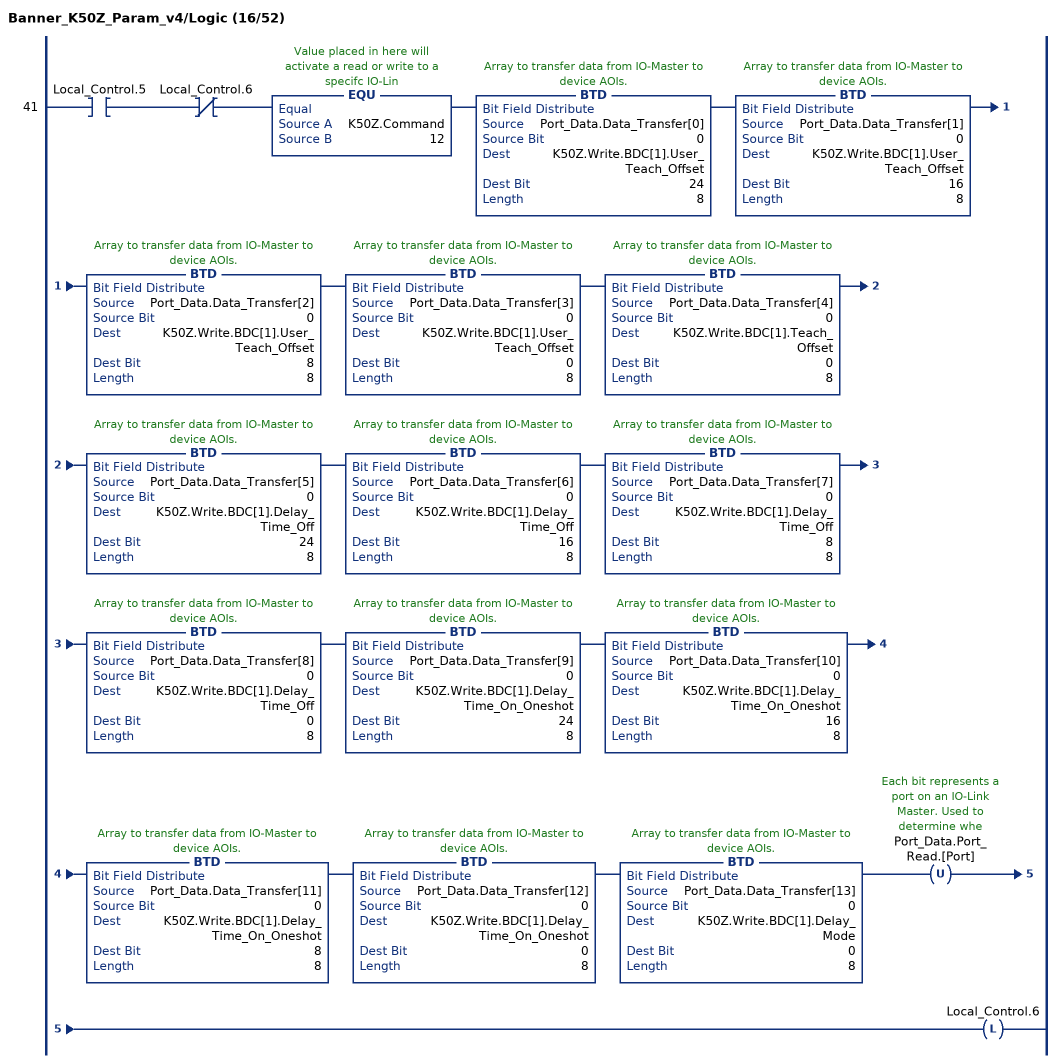
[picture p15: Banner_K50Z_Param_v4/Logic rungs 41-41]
   41: XIC(Local_Control.5)XIO(Local_Control.6)EQU(K50Z.Command,12)BTD(Port_Data.Data_Transfer[0],0,K50Z.Write.BDC[1].User_Teach_Offset,24,8)BTD(Port_Data.Data_Transfer[1],0,K50Z.Write.BDC[1].User_Teach_Offset,16,8)BTD(Port_Data.Data_Transfer[2],0,K50Z.Write.BDC[1].User_Teach_Offset,8,8)BTD(Port_Data.Data_Transfer[3],0,K50Z.Write.BDC[1].User_Teach_Offset,0,8)BTD(Port_Data.Data_Transfer[4],0,K50Z.Write.BDC[1].Teach_Offset,0,8)BTD(Port_Data.Data_Transfer[5],0,K50Z.Write.BDC[1].Delay_Time_Off,24,8)BTD(Port_Data.Data_Transfer[6],0,K50Z.Write.BDC[1].Delay_Time_Off,16,8)BTD(Port_Data.Data_Transfer[7],0,K50Z.Write.BDC[1].Delay_Time_Off,8,8)BTD(Port_Data.Data_Transfer[8],0,K50Z.Write.BDC[1].Delay_Time_Off,0,8)BTD(Port_Data.Data_Transfer[9],0,K50Z.Write.BDC[1].Delay_Time_On_Oneshot,24,8)BTD(Port_Data.Data_Transfer[10],0,K50Z.Write.BDC[1].Delay_Time_On_Oneshot,16,8)BTD(Port_Data.Data_Transfer[11],0,K50Z.Write.BDC[1].Delay_Time_On_Oneshot,8,8)BTD(Port_Data.Data_Transfer[12],0,K50Z.Write.BDC[1].Delay_Time_On_Oneshot,0,8)BTD(Port_Data.Data_Transfer[13],0,K50Z.Write.BDC[1].Delay_Mode,0,8)OTU(Port_Data.Port_Read.[Port])OTL(Local_Control.6);
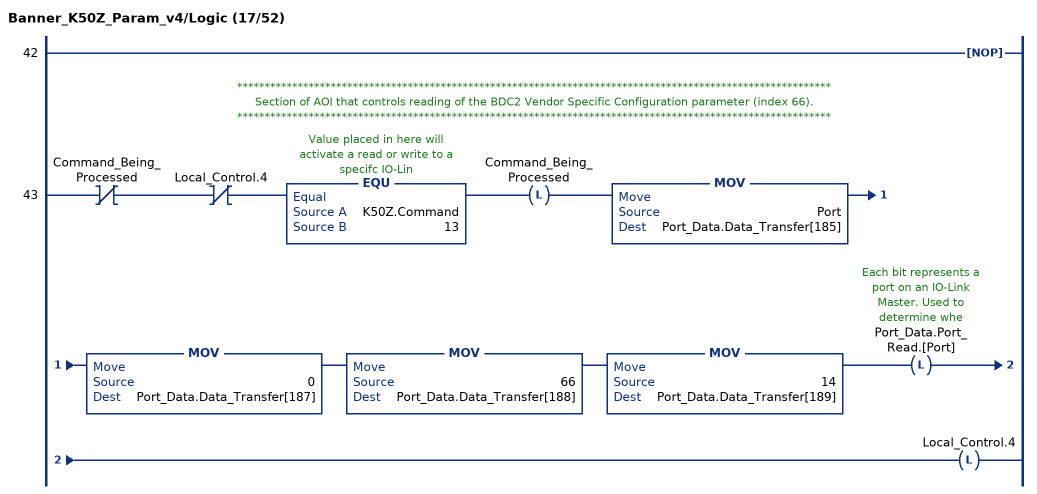
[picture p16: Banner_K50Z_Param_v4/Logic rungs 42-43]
   42: NOP();
   // ************************************************************************************************************
   // Section of AOI that controls reading of the BDC2 Vendor Specific Configuration parameter (index 66).
   // ************************************************************************************************************
   43: XIO(Command_Being_Processed)XIO(Local_Control.4)EQU(K50Z.Command,13)OTL(Command_Being_Processed)MOV(Port,Port_Data.Data_Transfer[185])MOV(0,Port_Data.Data_Transfer[187])MOV(66,Port_Data.Data_Transfer[188])MOV(14,Port_Data.Data_Transfer[189])OTL(Port_Data.Port_Read.[Port])OTL(Local_Control.4);
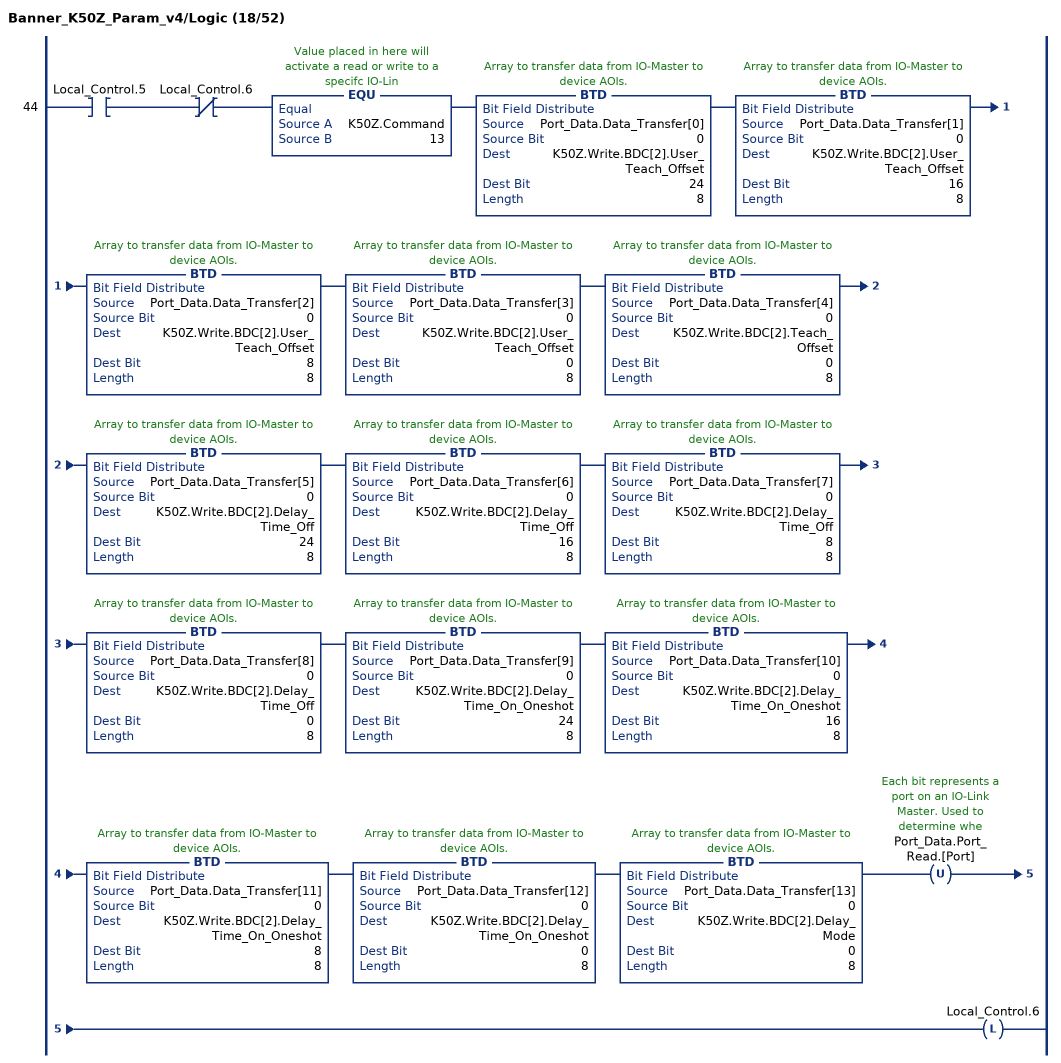
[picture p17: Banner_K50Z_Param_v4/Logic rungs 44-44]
   44: XIC(Local_Control.5)XIO(Local_Control.6)EQU(K50Z.Command,13)BTD(Port_Data.Data_Transfer[0],0,K50Z.Write.BDC[2].User_Teach_Offset,24,8)BTD(Port_Data.Data_Transfer[1],0,K50Z.Write.BDC[2].User_Teach_Offset,16,8)BTD(Port_Data.Data_Transfer[2],0,K50Z.Write.BDC[2].User_Teach_Offset,8,8)BTD(Port_Data.Data_Transfer[3],0,K50Z.Write.BDC[2].User_Teach_Offset,0,8)BTD(Port_Data.Data_Transfer[4],0,K50Z.Write.BDC[2].Teach_Offset,0,8)BTD(Port_Data.Data_Transfer[5],0,K50Z.Write.BDC[2].Delay_Time_Off,24,8)BTD(Port_Data.Data_Transfer[6],0,K50Z.Write.BDC[2].Delay_Time_Off,16,8)BTD(Port_Data.Data_Transfer[7],0,K50Z.Write.BDC[2].Delay_Time_Off,8,8)BTD(Port_Data.Data_Transfer[8],0,K50Z.Write.BDC[2].Delay_Time_Off,0,8)BTD(Port_Data.Data_Transfer[9],0,K50Z.Write.BDC[2].Delay_Time_On_Oneshot,24,8)BTD(Port_Data.Data_Transfer[10],0,K50Z.Write.BDC[2].Delay_Time_On_Oneshot,16,8)BTD(Port_Data.Data_Transfer[11],0,K50Z.Write.BDC[2].Delay_Time_On_Oneshot,8,8)BTD(Port_Data.Data_Transfer[12],0,K50Z.Write.BDC[2].Delay_Time_On_Oneshot,0,8)BTD(Port_Data.Data_Transfer[13],0,K50Z.Write.BDC[2].Delay_Mode,0,8)OTU(Port_Data.Port_Read.[Port])OTL(Local_Control.6);
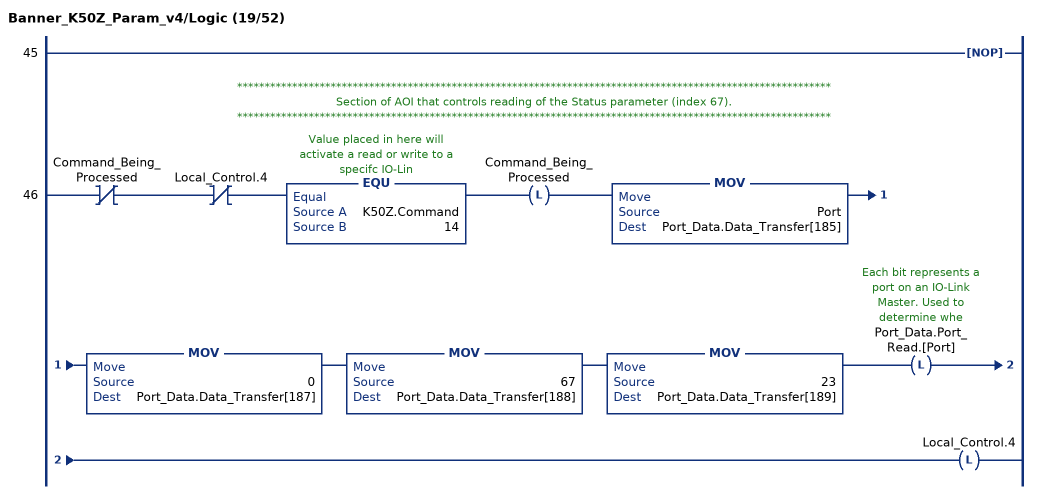
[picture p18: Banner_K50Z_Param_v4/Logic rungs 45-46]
   45: NOP();
   // ************************************************************************************************************
   // Section of AOI that controls reading of the Status parameter (index 67).
   // ************************************************************************************************************
   46: XIO(Command_Being_Processed)XIO(Local_Control.4)EQU(K50Z.Command,14)OTL(Command_Being_Processed)MOV(Port,Port_Data.Data_Transfer[185])MOV(0,Port_Data.Data_Transfer[187])MOV(67,Port_Data.Data_Transfer[188])MOV(23,Port_Data.Data_Transfer[189])OTL(Port_Data.Port_Read.[Port])OTL(Local_Control.4);
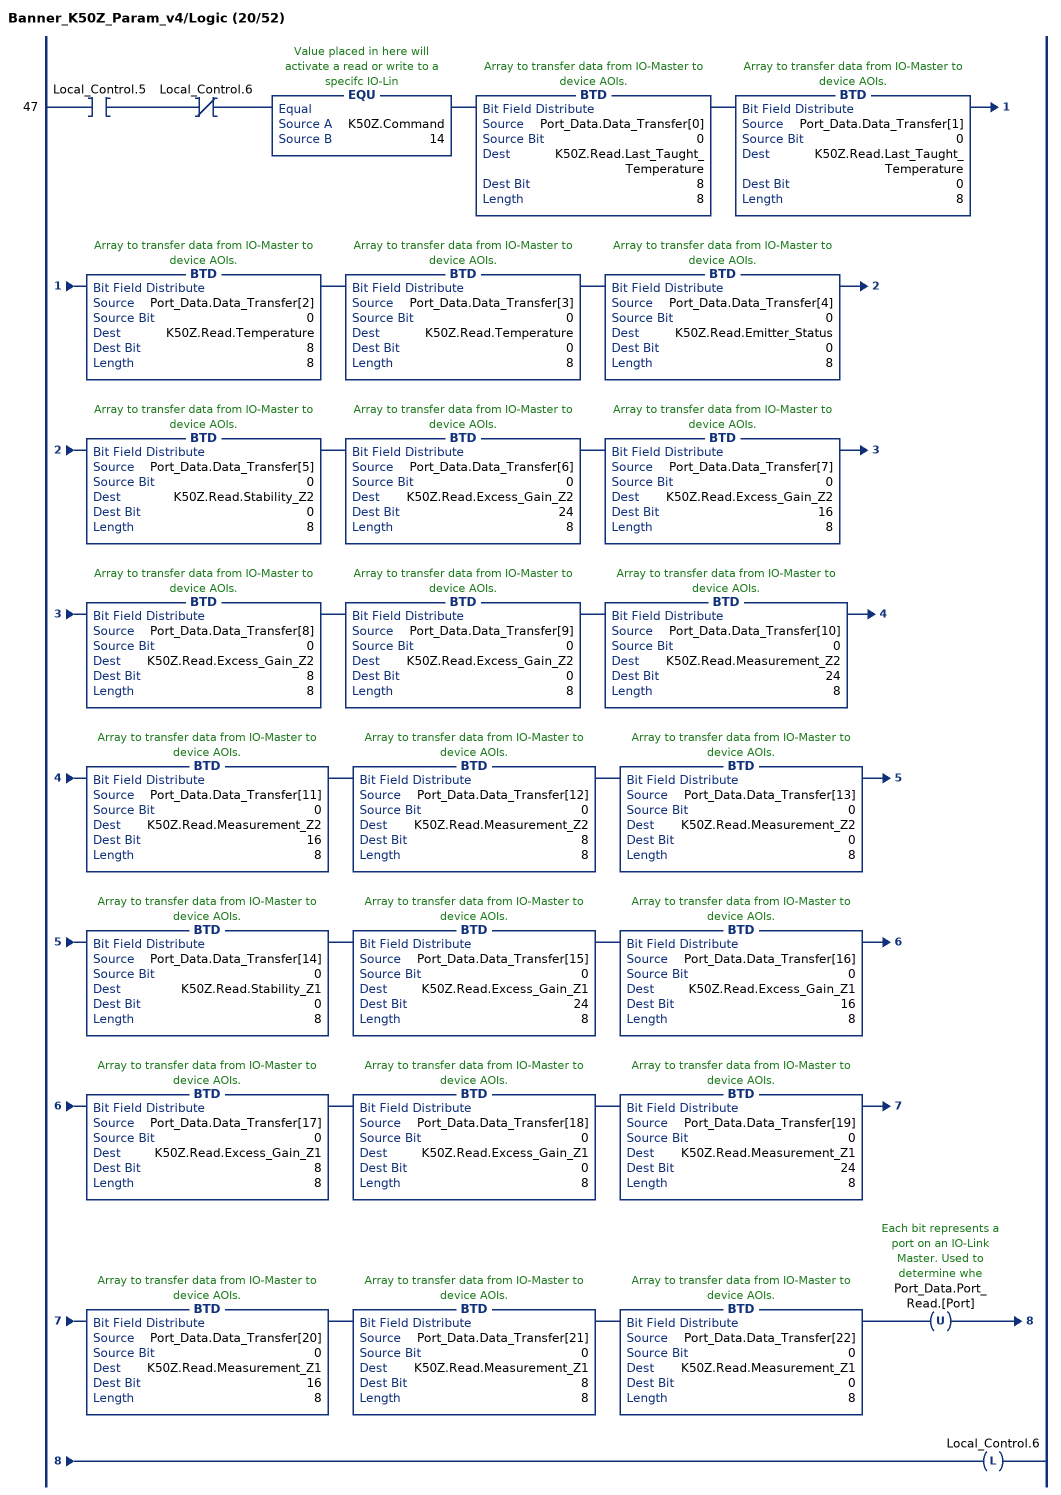
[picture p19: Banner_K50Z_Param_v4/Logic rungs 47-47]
   47: XIC(Local_Control.5)XIO(Local_Control.6)EQU(K50Z.Command,14)BTD(Port_Data.Data_Transfer[0],0,K50Z.Read.Last_Taught_Temperature,8,8)BTD(Port_Data.Data_Transfer[1],0,K50Z.Read.Last_Taught_Temperature,0,8)BTD(Port_Data.Data_Transfer[2],0,K50Z.Read.Temperature,8,8)BTD(Port_Data.Data_Transfer[3],0,K50Z.Read.Temperature,0,8)BTD(Port_Data.Data_Transfer[4],0,K50Z.Read.Emitter_Status,0,8)BTD(Port_Data.Data_Transfer[5],0,K50Z.Read.Stability_Z2,0,8)BTD(Port_Data.Data_Transfer[6],0,K50Z.Read.Excess_Gain_Z2,24,8)BTD(Port_Data.Data_Transfer[7],0,K50Z.Read.Excess_Gain_Z2,16,8)BTD(Port_Data.Data_Transfer[8],0,K50Z.Read.Excess_Gain_Z2,8,8)BTD(Port_Data.Data_Transfer[9],0,K50Z.Read.Excess_Gain_Z2,0,8)BTD(Port_Data.Data_Transfer[10],0,K50Z.Read.Measurement_Z2,24,8)BTD(Port_Data.Data_Transfer[11],0,K50Z.Read.Measurement_Z2,16,8)BTD(Port_Data.Data_Transfer[12],0,K50Z.Read.Measurement_Z2,8,8)BTD(Port_Data.Data_Transfer[13],0,K50Z.Read.Measurement_Z2,0,8)BTD(Port_Data.Data_Transfer[14],0,K50Z.Read.Stability_Z1,0,8)BTD(Port_Data.Data_Transfer[15],0,K50Z.Read.Excess_Gain_Z1,24,8)BTD(Port_Data.Data_Transfer[16],0,K50Z.Read.Excess_Gain_Z1,16,8)BTD(Port_Data.Data_Transfer[17],0,K50Z.Read.Excess_Gain_Z1,8,8)BTD(Port_Data.Data_Transfer[18],0,K50Z.Read.Excess_Gain_Z1,0,8)BTD(Port_Data.Data_Transfer[19],0,K50Z.Read.Measurement_Z1,24,8)BTD(Port_Data.Data_Transfer[20],0,K50Z.Read.Measurement_Z1,16,8)BTD(Port_Data.Data_Transfer[21],0,K50Z.Read.Measurement_Z1,8,8)BTD(Port_Data.Data_Transfer[22],0,K50Z.Read.Measurement_Z1,0,8)OTU(Port_Data.Port_Read.[Port])OTL(Local_Control.6);
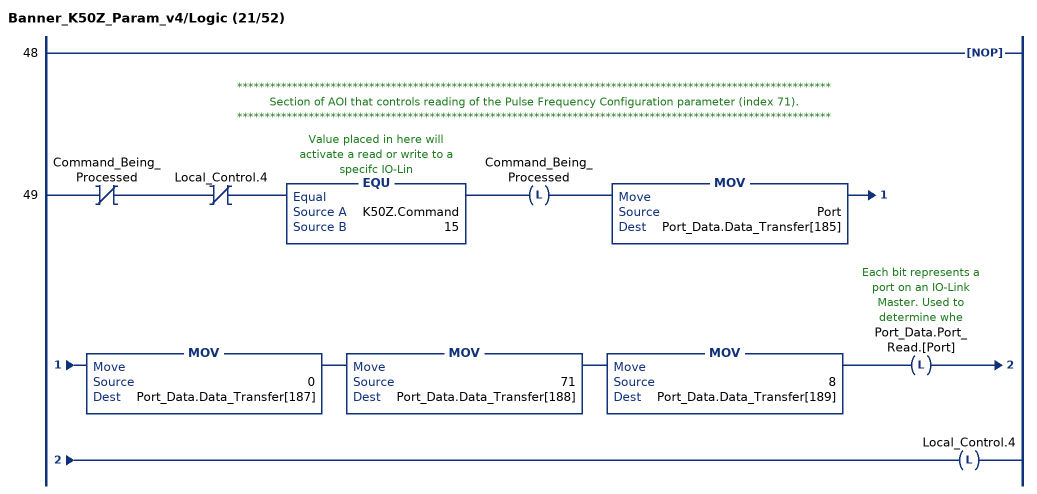
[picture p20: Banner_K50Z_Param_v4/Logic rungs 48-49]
   48: NOP();
   // ************************************************************************************************************
   // Section of AOI that controls reading of the Pulse Frequency Configuration parameter (index 71).
   // ************************************************************************************************************
   49: XIO(Command_Being_Processed)XIO(Local_Control.4)EQU(K50Z.Command,15)OTL(Command_Being_Processed)MOV(Port,Port_Data.Data_Transfer[185])MOV(0,Port_Data.Data_Transfer[187])MOV(71,Port_Data.Data_Transfer[188])MOV(8,Port_Data.Data_Transfer[189])OTL(Port_Data.Port_Read.[Port])OTL(Local_Control.4);
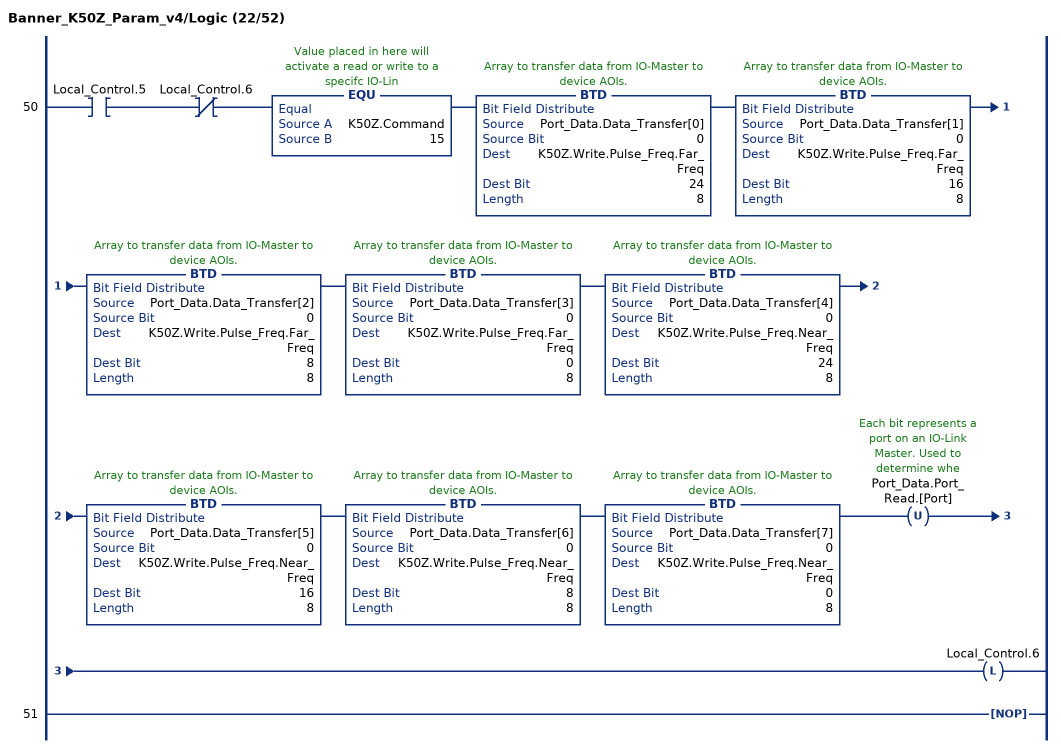
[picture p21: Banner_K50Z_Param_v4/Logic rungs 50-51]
   50: XIC(Local_Control.5)XIO(Local_Control.6)EQU(K50Z.Command,15)BTD(Port_Data.Data_Transfer[0],0,K50Z.Write.Pulse_Freq.Far_Freq,24,8)BTD(Port_Data.Data_Transfer[1],0,K50Z.Write.Pulse_Freq.Far_Freq,16,8)BTD(Port_Data.Data_Transfer[2],0,K50Z.Write.Pulse_Freq.Far_Freq,8,8)BTD(Port_Data.Data_Transfer[3],0,K50Z.Write.Pulse_Freq.Far_Freq,0,8)BTD(Port_Data.Data_Transfer[4],0,K50Z.Write.Pulse_Freq.Near_Freq,24,8)BTD(Port_Data.Data_Transfer[5],0,K50Z.Write.Pulse_Freq.Near_Freq,16,8)BTD(Port_Data.Data_Transfer[6],0,K50Z.Write.Pulse_Freq.Near_Freq,8,8)BTD(Port_Data.Data_Transfer[7],0,K50Z.Write.Pulse_Freq.Near_Freq,0,8)OTU(Port_Data.Port_Read.[Port])OTL(Local_Control.6);
   51: NOP();
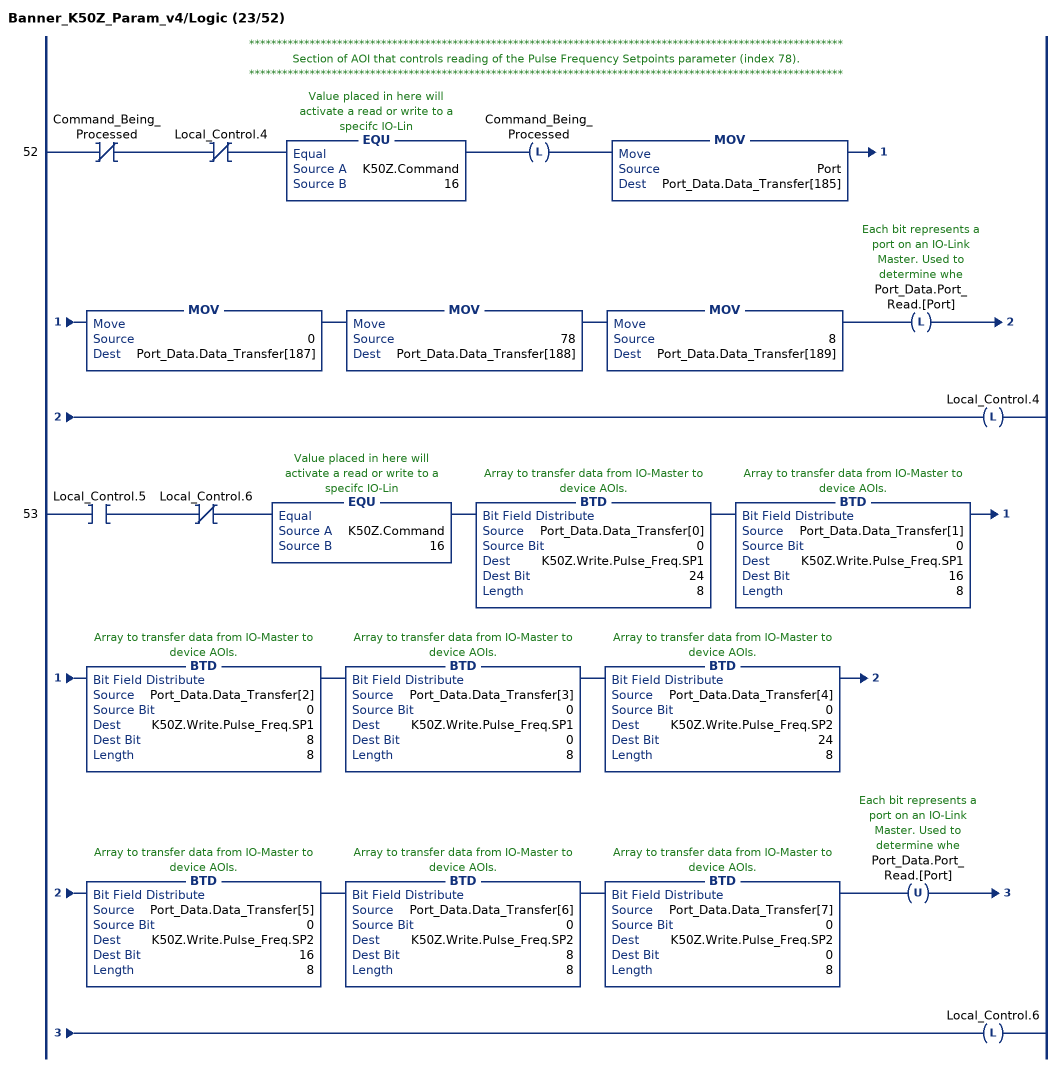
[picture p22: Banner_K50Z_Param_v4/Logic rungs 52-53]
   // ************************************************************************************************************
   // Section of AOI that controls reading of the Pulse Frequency Setpoints parameter (index 78).
   // ************************************************************************************************************
   52: XIO(Command_Being_Processed)XIO(Local_Control.4)EQU(K50Z.Command,16)OTL(Command_Being_Processed)MOV(Port,Port_Data.Data_Transfer[185])MOV(0,Port_Data.Data_Transfer[187])MOV(78,Port_Data.Data_Transfer[188])MOV(8,Port_Data.Data_Transfer[189])OTL(Port_Data.Port_Read.[Port])OTL(Local_Control.4);
   53: XIC(Local_Control.5)XIO(Local_Control.6)EQU(K50Z.Command,16)BTD(Port_Data.Data_Transfer[0],0,K50Z.Write.Pulse_Freq.SP1,24,8)BTD(Port_Data.Data_Transfer[1],0,K50Z.Write.Pulse_Freq.SP1,16,8)BTD(Port_Data.Data_Transfer[2],0,K50Z.Write.Pulse_Freq.SP1,8,8)BTD(Port_Data.Data_Transfer[3],0,K50Z.Write.Pulse_Freq.SP1,0,8)BTD(Port_Data.Data_Transfer[4],0,K50Z.Write.Pulse_Freq.SP2,24,8)BTD(Port_Data.Data_Transfer[5],0,K50Z.Write.Pulse_Freq.SP2,16,8)BTD(Port_Data.Data_Transfer[6],0,K50Z.Write.Pulse_Freq.SP2,8,8)BTD(Port_Data.Data_Transfer[7],0,K50Z.Write.Pulse_Freq.SP2,0,8)OTU(Port_Data.Port_Read.[Port])OTL(Local_Control.6);
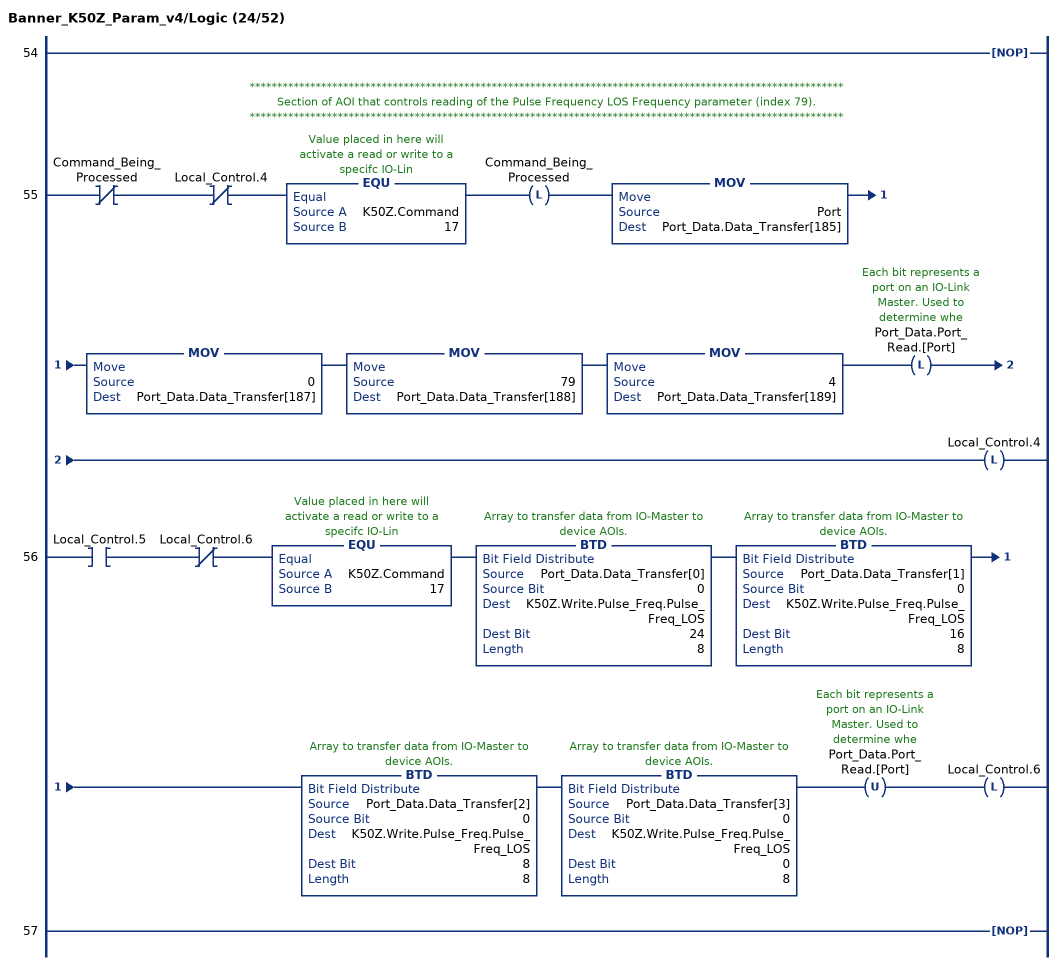
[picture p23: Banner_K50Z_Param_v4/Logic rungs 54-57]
   54: NOP();
   // ************************************************************************************************************
   // Section of AOI that controls reading of the Pulse Frequency LOS Frequency parameter (index 79).
   // ************************************************************************************************************
   55: XIO(Command_Being_Processed)XIO(Local_Control.4)EQU(K50Z.Command,17)OTL(Command_Being_Processed)MOV(Port,Port_Data.Data_Transfer[185])MOV(0,Port_Data.Data_Transfer[187])MOV(79,Port_Data.Data_Transfer[188])MOV(4,Port_Data.Data_Transfer[189])OTL(Port_Data.Port_Read.[Port])OTL(Local_Control.4);
   56: XIC(Local_Control.5)XIO(Local_Control.6)EQU(K50Z.Command,17)BTD(Port_Data.Data_Transfer[0],0,K50Z.Write.Pulse_Freq.Pulse_Freq_LOS,24,8)BTD(Port_Data.Data_Transfer[1],0,K50Z.Write.Pulse_Freq.Pulse_Freq_LOS,16,8)BTD(Port_Data.Data_Transfer[2],0,K50Z.Write.Pulse_Freq.Pulse_Freq_LOS,8,8)BTD(Port_Data.Data_Transfer[3],0,K50Z.Write.Pulse_Freq.Pulse_Freq_LOS,0,8)OTU(Port_Data.Port_Read.[Port])OTL(Local_Control.6);
   57: NOP();
